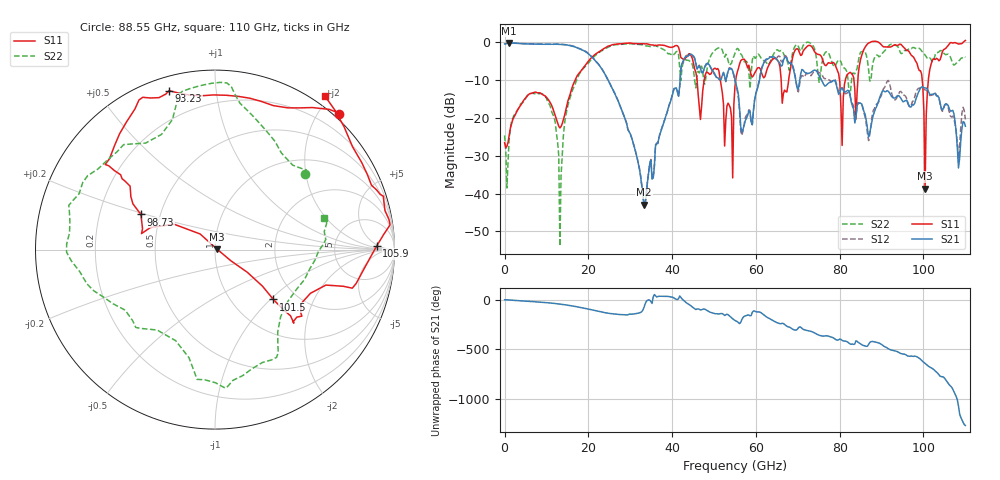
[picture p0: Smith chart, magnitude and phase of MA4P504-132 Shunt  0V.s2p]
!Keysight Technologies,N5247B,US61255204,A.15.70.20
!Date: Friday, October 21, 2022 14:50:30
!Correction: S11(C  4-Port  )
!S31(C  4-Port  )
!S13(C  4-Port  )
!S33(C  4-Port  )
!S2P File: Measurements: S11, S31, S13, S33:
# Hz S  dB  R 50
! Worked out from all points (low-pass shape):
!   401 points, 10 MHz to 110 GHz, reference 50 ohm
!   highest |S21| = -0.20 dB at 1.11 GHz (marker M1); lowest = -42.9 dB at 33.28 GHz (marker M2)
!   |S21| within 3 dB of the highest: start of sweep to 20.13 GHz; 44.24 GHz to 44.58 GHz (338.7 MHz wide, 0.763 % of centre)
!   lowest |S11| = -38.7 dB at 100.4 GHz (marker M3), VSWR 1.02, Z = 51.1 + j0.267 ohm
!   |S11| at or under -10 dB: start of sweep to 16.87 GHz; 45.95 GHz to 47.66 GHz (1.707 GHz wide, 3.65 % of centre); 51.49 GHz to 55.19 GHz (3.695 GHz wide, 6.93 % of centre)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
!   |S22| runs from -53.9 to 0.0 dB; largest |S21 - S12| = 0.25
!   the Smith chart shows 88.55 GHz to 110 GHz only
!   S11 on the Smith chart (normalised r, x): 88.55 GHz: -0.08, +2.27; 93.23 GHz: 0.06, +0.75; 98.73 GHz: 0.39, +0.19; 101.5 GHz: 1.53, -1.04; 105.9 GHz: 18, +4; 110 GHz: -0.12, +1.95
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1e7  -26.54 2.6  -0.49 -0.2  -0.50 -0.1  -24.64 -0.7
1.1099e9  -24.52 68.2  -0.20 -2.8  -0.19 -2.6  -25.30 104.1
9.084175e9  -13.87 75.8  -0.57 -26.0  -0.54 -25.7  -13.71 57.4
1.32088e10  -22.66 130.4  -0.61 -43.7  -0.56 -43.1  -53.90 -4.4
1.843332e10  -7.31 173.6  -2.01 -79.8  -1.96 -79.7  -7.40 -162.8
3.328198e10  -0.45 118.3  -42.92 -77.2  -42.82 -77.6  -0.80 122.2
3.685665e10  -0.76 117.4  -25.29 35.7  -25.12 35.5  -1.32 126.4
4.428098e10  -3.12 24.2  -3.17 -54.8  -3.33 -55.2  -5.13 74.9
4.84056e10  -7.96 -167.4  -5.62 -109.7  -5.62 -109.7  -6.64 135.4
5.5005e10  -11.59 -107.9  -10.00 151.5  -10.25 149.7  -2.97 168.1
5.692982e10  -4.52 -112.3  -23.01 -178.1  -23.29 -164.9  -4.30 156.9
6.6004e10  -9.59 -36.9  -6.35 118.3  -5.02 123.1  -2.21 48.3
7.342832e10  -1.36 138.3  -7.74 37.4  -8.44 35.9  -0.69 108.7
7.975275e10  -8.37 -164.5  -13.82 -43.3  -13.33 -44.1  -4.72 -142.6
8.855195e10  0.22 47.5  -17.60 -66.4  -16.74 -48.5  -3.68 40.3
9.185165e10  -1.29 90.5  -13.36 -138.9  -10.71 -132.9  -0.80 84.3
9.322652e10  -0.71 106.1  -14.75 -156.0  -15.27 -153.7  -0.82 98.3
9.872602e10  -6.80 154.6  -13.43 137.7  -12.24 137.8  -1.65 177.8
1.003759e11  -38.68 12.9  -12.12 79.1  -12.62 81.1  -3.44 -156.6
1.014758e11  -7.38 -40.5  -13.78 43.0  -14.10 49.2  -4.17 -135.5
1.058754e11  -0.90 1.3  -16.72 -121.9  -17.24 -124.4  -3.20 -60.3
1.1e11  0.44 54.3  -22.23 173.3  -20.43 174.9  -4.00 16.1
